(* Logix 5000 AddOnInstructionDefinition export B256_ADD; software revision 30.00 *)

ADD_ON_INSTRUCTION B256_ADD   (* revision 1.0 20170916, vendor Kenneth A. Fischer *)
// c3=c1+c2 with no reduction
// Revision note:
// Rev1.0: 20170916 - Initial Release
VAR_IN_OUT
   Inp_C1 : DINT[22]; {required}
   Inp_C2 : DINT[22]; {required}
   Out_C3 : DINT[22]; {required}
END_VAR
VAR
   i : INT;
END_VAR

ROUTINE Logic   (* ladder *)
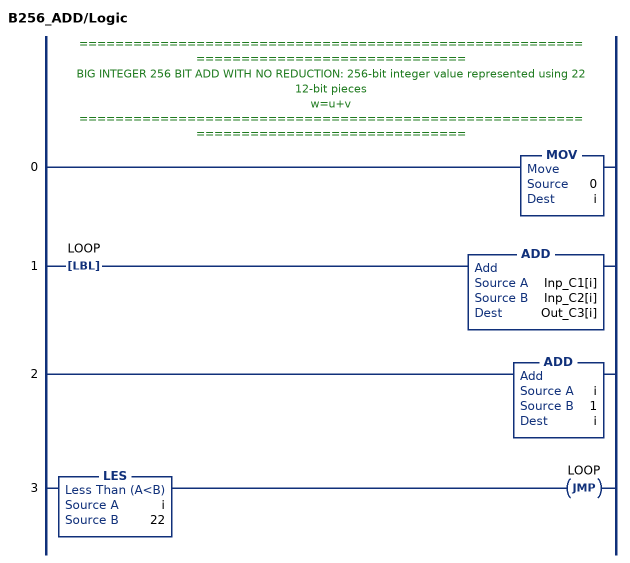
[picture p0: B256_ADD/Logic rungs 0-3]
   // ======================================================================================
   // BIG INTEGER 256 BIT ADD WITH NO REDUCTION: 256-bit integer value represented using 22 12-bit pieces
   // w=u+v
   // ======================================================================================
   0: MOV(0,i);
   1: LBL(LOOP)ADD(Inp_C1[i],Inp_C2[i],Out_C3[i]);
   2: ADD(i,1,i);
   3: LES(i,22)JMP(LOOP);
END_ROUTINE
END_ADD_ON_INSTRUCTION
